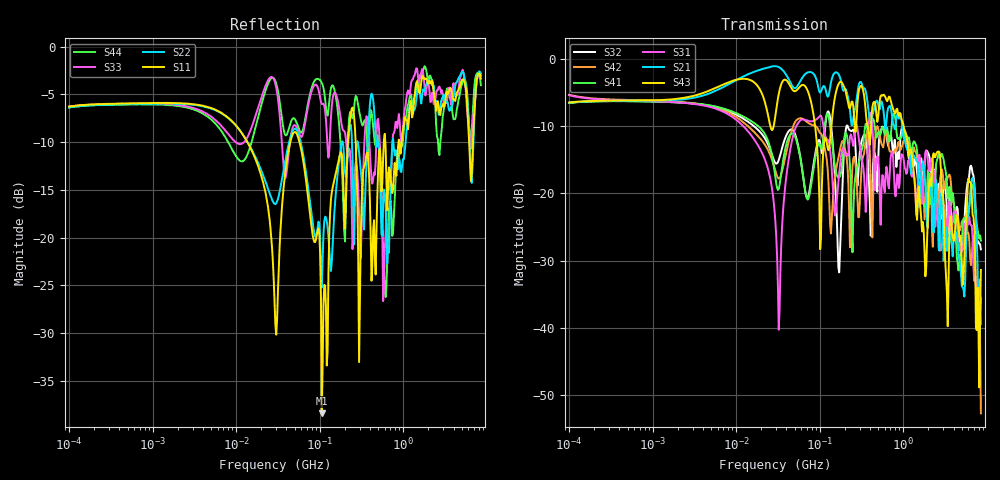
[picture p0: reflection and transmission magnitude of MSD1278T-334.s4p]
# MHz S MA R 50
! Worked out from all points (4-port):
!   498 points, 100 kHz to 8.5 GHz, reference 50 ohm
!   strongest paths, dB at 100 kHz, 1.698 MHz, 29.49 MHz, 500.7 MHz, 8.5 GHz:
!     S43: -6.5, -6.0, -8.4, -8.6, -31.4
!     S21: -6.5, -6.1, -1.0, -6.7, -35.6
!     S31: -5.4, -6.4, -24.3, -14.8, -39.5
!     S41: -6.5, -6.4, -17.6, -10.8, -27.0
!     S42: -5.3, -6.3, -16.7, -10.3, -52.8
!     S32: -6.5, -6.4, -15.5, -15.2, -28.3
!   lowest |S11| = -38.4 dB at 105.9 MHz (marker M1), VSWR 1.02, Z = 50 - j1.2 ohm
!   |S11| at or under -10 dB: 269.2 MHz to 585.7 MHz (316.6 MHz wide, 74.1 % of centre); 609.8 MHz to 879.2 MHz (269.4 MHz wide, 36.2 % of centre); 6.153 GHz to 6.834 GHz (681.7 MHz wide, 10.5 % of centre)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
0.1  0.4847 13.8  0.4746 14.7  0.5391 -13.5  0.473 -166.5
     0.4746 14.7  0.4793 13.8  0.4727 -166.4  0.5429 -13.4
     0.5391 -13.5  0.4727 -166.4  0.484 13.9  0.4756 14.7
     0.473 -166.5  0.5429 -13.4  0.4756 14.7  0.4793 13.9
32.31038  0.06855 42.1  0.8744 -12.2  0.009645 38.1  0.1079 41.4
          0.8744 -12.2  0.1652 1.6  0.1772 56.2  0.1289 -167.2
          0.009645 38.1  0.1772 56.2  0.4916 -44.7  0.5505 13.4
          0.1079 41.4  0.1289 -167.2  0.5505 13.4  0.554 -25.0
105.9488  0.01202 -90.5  0.5964 -24.4  0.367 -21.8  0.2154 63.5
          0.5964 -24.4  0.05479 -9.8  0.2017 50.2  0.2729 -20.1
          0.367 -21.8  0.2017 50.2  0.4999 -35.7  0.109 37.6
          0.2154 63.5  0.2729 -20.1  0.109 37.6  0.6446 -35.2
614.9063  0.2984 -69.2  0.302 -92.6  0.135 -49.8  0.2804 -50.6
          0.302 -92.6  0.1515 -89.4  0.2865 -55.9  0.2854 -50.9
          0.135 -49.8  0.2865 -55.9  0.1041 -21.8  0.5167 -90.9
          0.2804 -50.6  0.2854 -50.9  0.5167 -90.9  0.04878 122.3
1840.304  0.6745 -157.9  0.1123 114.1  0.2028 177.3  0.07769 163.1
          0.1123 114.1  0.6169 -149.2  0.1947 -177.0  0.08194 159.9
          0.2028 177.3  0.1947 -177.0  0.5541 -165.7  0.02413 32.9
          0.07769 163.1  0.08194 159.9  0.02413 32.9  0.7795 -162.7
3568.796  0.5952 11.9  0.05166 -120.8  0.08676 1.0  0.1123 -17.6
          0.05166 -120.8  0.4607 9.9  0.09372 20.2  0.1382 -13.7
          0.08676 1.0  0.09372 20.2  0.6094 3.8  0.05244 130.4
          0.1123 -17.6  0.1382 -13.7  0.05244 130.4  0.5401 -9.9
8500  0.6792 -57.7  0.01662 -36.7  0.01063 -67.7  0.04457 -154.9
      0.01662 -36.7  0.7208 -54.5  0.03833 -120.7  0.0023 -9.5
      0.01063 -67.7  0.03833 -120.7  0.7046 -58.0  0.02693 3.2
      0.04457 -154.9  0.0023 -9.5  0.02693 3.2  0.6273 -59.8
